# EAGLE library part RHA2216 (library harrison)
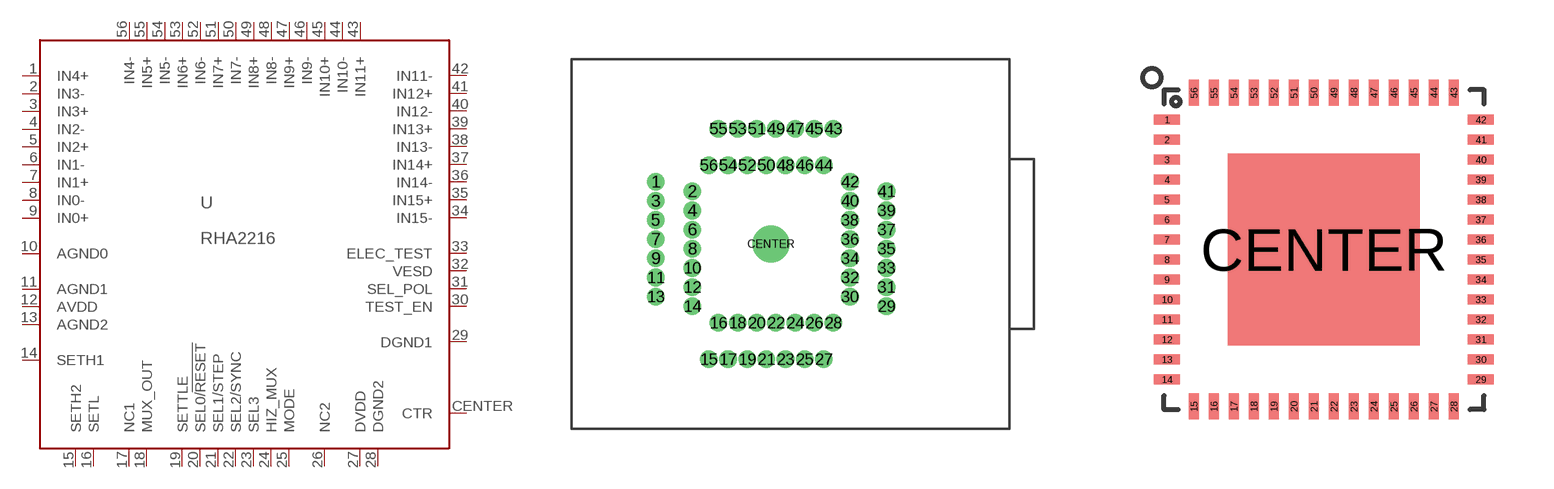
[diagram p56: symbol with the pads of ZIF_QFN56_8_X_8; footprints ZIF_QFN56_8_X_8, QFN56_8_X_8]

Designator prefix U

## RHA2216ZIF  [ZIF_QFN56_8_X_8]
1  IN4+  in
2  IN3-  in
3  IN3+  in
4  IN2-  in
5  IN2+  in
6  IN1-  in
7  IN1+  in
8  IN0-  in
9  IN0+  in
10  AGND0  in
11  AGND1  pwr
12  AVDD  pwr
13  AGND2  pwr
14  SETH1  pas
15  SETH2  pas
16  SETL  pas
17  NC1  nc
18  MUX_OUT  hiz
19  SETTLE  in
20  SEL0/!RESET!  in
21  SEL1/STEP  in
22  SEL2/SYNC
23  SEL3
24  HIZ_MUX  in
25  MODE  in
26  NC2  nc
27  DVDD  pwr
28  DGND2  pwr
29  DGND1  pwr
30  TEST_EN  in
31  SEL_POL  in
32  VESD  pwr
33  ELEC_TEST  in
34  IN15-  in
35  IN15+  in
36  IN14-  in
37  IN14+  in
38  IN13-  in
39  IN13+  in
40  IN12-  in
41  IN12+  in
42  IN11-  in
43  IN11+  in
44  IN10-  in
45  IN10+  in
46  IN9-  in
47  IN9+  in
48  IN8-  in
49  IN8+  in
50  IN7-  in
51  IN7+  in
52  IN6-  in
53  IN6+  in
54  IN5-  in
55  IN5+  in
56  IN4-  in
CENTER  CTR  pwr

## RHA2216QFN  [QFN56_8_X_8]
Pads as for ZIF_QFN56_8_X_8

## Footprint ZIF_QFN56_8_X_8 (pad centres in mm)
drill 0.41 pad 0.813: 1 -6.02,3.251; 2 -4.115,2.751; 3 -6.02,2.25; 4 -4.115,1.75; 5 -6.02,1.25; 6 -4.115,0.752; 7 -6.02,0.249; 8 -4.115,-0.249; 9 -6.02,-0.749; 10 -4.115,-1.25; 11 -6.02,-1.75; 12 -4.115,-2.25; 13 -6.02,-2.751; 14 -4.115,-3.251; 15 -3.251,-6.02; 16 -2.751,-4.115; 17 -2.25,-6.02; 18 -1.75,-4.115; 19 -1.25,-6.02; 20 -0.752,-4.115; 21 -0.249,-6.02; 22 0.249,-4.115; 23 0.749,-6.02; 24 1.25,-4.115; 25 1.75,-6.02; 26 2.25,-4.115; 27 2.751,-6.02; 28 3.251,-4.115; 29 6.02,-3.251; 30 4.115,-2.751; 31 6.02,-2.25; 32 4.115,-1.75; 33 6.02,-1.25; 34 4.115,-0.752; 35 6.02,-0.249; 36 4.115,0.249; 37 6.02,0.749; 38 4.115,1.25; 39 6.02,1.75; 40 4.115,2.25; 41 6.02,2.751; 42 4.115,3.251; 43 3.251,6.02; 44 2.751,4.115; 45 2.25,6.02; 46 1.75,4.115; 47 1.25,6.02; 48 0.752,4.115; 49 0.249,6.02; 50 -0.249,4.115; 51 -0.749,6.02; 52 -1.25,4.115; 53 -1.75,6.02; 54 -2.25,4.115; 55 -2.751,6.02; 56 -3.251,4.115
drill 1.02 pad 1.93: CENTER 0,0

## Footprint QFN56_8_X_8 (pad centres in mm)
smd 0.65 x 0.25: 1 -3.925,3.25; 2 -3.925,2.75; 3 -3.925,2.25; 4 -3.925,1.75; 5 -3.925,1.25; 6 -3.925,0.75; 7 -3.925,0.25; 8 -3.925,-0.25; 9 -3.925,-0.75; 10 -3.925,-1.25; 11 -3.925,-1.75; 12 -3.925,-2.25; 13 -3.925,-2.75; 14 -3.925,-3.25; 29 3.925,-3.25; 30 3.925,-2.75; 31 3.925,-2.25; 32 3.925,-1.75; 33 3.925,-1.25; 34 3.925,-0.75; 35 3.925,-0.25; 36 3.925,0.25; 37 3.925,0.75; 38 3.925,1.25; 39 3.925,1.75; 40 3.925,2.25; 41 3.925,2.75; 42 3.925,3.25
smd 0.25 x 0.65: 15 -3.25,-3.925; 16 -2.75,-3.925; 17 -2.25,-3.925; 18 -1.75,-3.925; 19 -1.25,-3.925; 20 -0.75,-3.925; 21 -0.25,-3.925; 22 0.25,-3.925; 23 0.75,-3.925; 24 1.25,-3.925; 25 1.75,-3.925; 26 2.25,-3.925; 27 2.75,-3.925; 28 3.25,-3.925; 43 3.25,3.925; 44 2.75,3.925; 45 2.25,3.925; 46 1.75,3.925; 47 1.25,3.925; 48 0.75,3.925; 49 0.25,3.925; 50 -0.25,3.925; 51 -0.75,3.925; 52 -1.25,3.925; 53 -1.75,3.925; 54 -2.25,3.925; 55 -2.75,3.925; 56 -3.25,3.925
smd 4.8 x 4.8: CENTER 0,0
